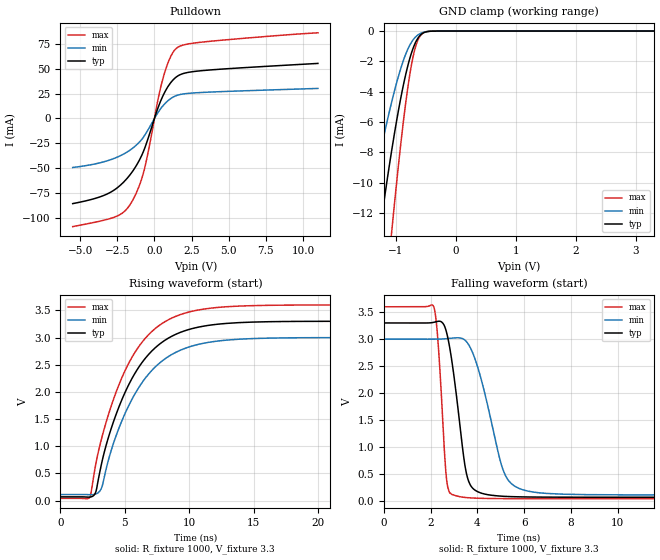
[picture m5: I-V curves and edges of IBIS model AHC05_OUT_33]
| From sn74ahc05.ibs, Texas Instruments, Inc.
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[Model]   AHC05_OUT_33
Model_type  Open_drain
Enable   Active-Low
Vref =   3.3
Rref =   1000
Cref =   50p
Vmeas =   1.65
| variable   typ   min   max
C_comp   2.19pF   1.62pF   2.51pF
| C_pulldown   4.35pF   2.48pF   6.72pF
| C_tri-state   2.19pF   1.62pF   2.51pF
[Temperature Range]   40   100   -40
| Ambient temperature   25   85   -40
[Voltage range]   3.3   3   3.6
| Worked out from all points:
|   slope of the pulldown table from 0 to 0.495 V, typ, clamps not added: 24.5 ohm
|   GND clamp passes 1 mA (typ) near -0.70 V on its own axis
|   rising waveform, R_fixture 1000, V_fixture 3.3: 20-80 % time 3.49ns typ, 3.54ns min, 3.44ns max; typ from 0.069 V to 3.3 V
|   falling waveform, R_fixture 1000, V_fixture 3.3: 20-80 % time 562ps typ, 962ps min, 289ps max; typ from 3.3 V to 0.069 V
[GND Clamp]
| AHC05_OUT_33
|   Voltage   I(typ)   I(min)   I(max)
-5.5V     -200.4mA   -131.5mA   -251.9mA
-1.515V   -20.84mA   -13.13mA   -33.21mA
-1.265V   -13.08mA   -8.076mA   -21.55mA
-1.07V    -7.831mA   -4.649mA   -13.18mA
-895mV    -3.917mA   -2.158mA   -6.583mA
-830mV    -2.733mA   -1.451mA   -4.512mA
-775mV    -1.883mA   -972.1uA   -3.005mA
-715mV    -1.142mA   -583uA     -1.697mA
-665mV    -683.2uA   -358.1uA   -926.1uA
-610mV    -342.4uA   -196.4uA   -406.4uA
-550mV    -137.1uA   -92.92uA   -137.6uA
3.3V      14.45nA    2.302nA    70.19nA
[Pulldown]
| AHC05_OUT_33
|   Voltage   I(typ)   I(min)   I(max)
-5.5V     -85.54mA   -49.27mA   -108.6mA
-3.025V   -74.71mA   -41.8mA    -100.7mA
-2.125V   -64.69mA   -36.15mA   -94.66mA
-1.53V    -54.33mA   -30.57mA   -83.84mA
-1.055V   -43.01mA   -24.39mA   -68.89mA
-695mV    -31.4mA    -17.77mA   -52.08mA
250mV     11.09mA    6.2mA      19.84mA
645mV     24.96mA    13.95mA    43.93mA
1.08V     35.65mA    19.81mA    61.78mA
1.5V      41.97mA    23.09mA    70.73mA
3.2V      48.02mA    26.12mA    76.68mA
11V       55.27mA    30.15mA    86.01mA
[Ramp]
| AHC05_OUT_33
| variable   typ   min   max
dV/dt_r   1.94/3.48E-09   1.73/3.54E-09   2.14/3.44E-09
dV/dt_f   1.96/5.70E-10   1.75/9.75E-10   2.16/2.98E-10
R_load = 1000
[Rising Waveform]
| AHC05_OUT_33
R_fixture =   1000
C_fixture =   0
L_fixture =   0
V_fixture =   3.3
V_fixture_min = 3
V_fixture_max = 3.6
|   Time   V(typ)   V(min)   V(max)
0s        68.53mV    111.3mV    41.42mV
2.21ns    63.89mV    109.2mV    44.37mV
2.64ns    110.7mV    114.5mV    539.6mV
3.195ns   686.4mV    237.9mV    1.146V
3.89ns    1.292V     886.6mV    1.706V
5.525ns   2.236V     1.854V     2.627V
7.345ns   2.811V     2.457V     3.164V
9.62ns    3.123V     2.797V     3.446V
16.1ns    3.291V     2.989V     3.592V
50ns      3.3V       3V         3.6V
[Falling Waveform]
| AHC05_OUT_33
R_fixture =   1000
C_fixture =   0
L_fixture =   0
V_fixture =   3.3
V_fixture_min = 3
V_fixture_max = 3.6
|   Time   V(typ)   V(min)   V(max)
0s        3.3V       3V         3.6V
2.135ns   3.312V     3V         3.594V
2.32ns    3.331V     3.001V     2.905V
2.7ns     3.087V     3.01V      328.2mV
3.305ns   1.197V     3.018V     74.06mV
3.51ns    551.4mV    2.962V     62.89mV
3.735ns   268.8mV    2.807V     55.56mV
5.185ns   84.58mV    485.5mV    42.8mV
6.415ns   72mV       162.8mV    41.65mV
50ns      68.53mV    111.3mV    41.42mV
